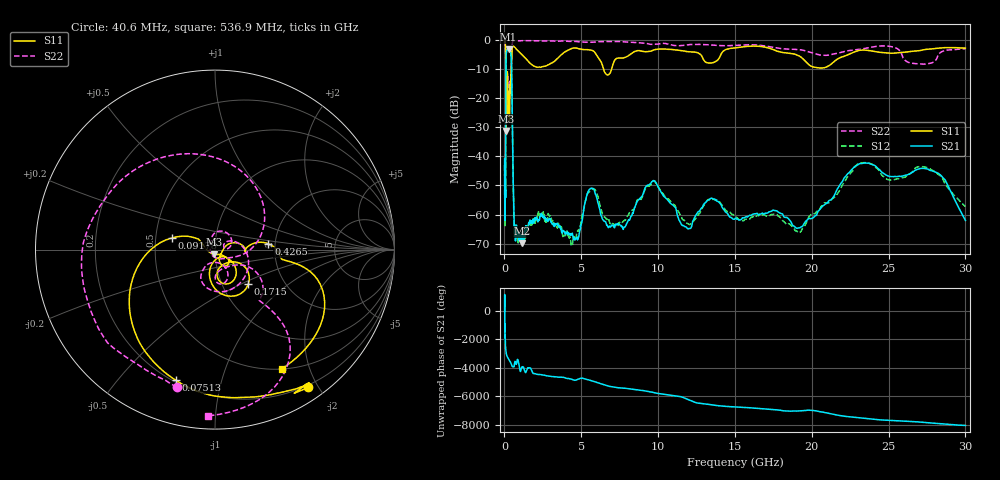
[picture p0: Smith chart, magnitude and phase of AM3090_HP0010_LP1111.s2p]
! Date/Time: Thu, Feb 28, 2019 1:56 PM
! Network Analyzer: Agilent Technologies E8364B Rev: A.07.50.67
! Sweep from 0.010 to 30.000 GHz, 1601 Points, Sweep Type: LOG
! Power Supply: 5.023 V, 0.002 A
# Hz S DB R 50
!freq MagS11 AngS11 MagS21 AngS21 MagS12 AngS12 MagS22 AngS22
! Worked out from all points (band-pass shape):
!   1601 points, 10 MHz to 30 GHz, reference 50 ohm
!   highest |S21| = -3.31 dB at 265.1 MHz (marker M1); lowest = -69.9 dB at 1.166 GHz (marker M2)
!   |S21| within 3 dB of the highest: 103.6 MHz to 441.7 MHz (338.1 MHz wide, 124 % of centre)
!   lowest |S11| = -31.3 dB at 99.92 MHz (marker M3), VSWR 1.06, Z = 49.5 - j2.64 ohm
!   |S11| at or under -10 dB: 90.68 MHz to 429.4 MHz (338.8 MHz wide, 130 % of centre); 6.451 GHz to 6.979 GHz (528.5 MHz wide, 7.87 % of centre)
!   |S22| runs from -31.6 to -0.2 dB; largest |S21 - S12| = 0.014
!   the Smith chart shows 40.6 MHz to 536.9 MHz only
!   S11 on the Smith chart (normalised r, x): 40.6 MHz: 0.17, -1.88; 75.13 MHz: 0.21, -0.72; 91.78 MHz: 0.61, +0.08; 171.5 MHz: 1.32, -0.55; 426.5 MHz: 1.84, +0.13; 536.9 MHz: 0.50, -1.59
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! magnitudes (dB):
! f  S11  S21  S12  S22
! 10 MHz  -0.3  -40.9  -43.0  -0.7
! 38.04 MHz  -0.5  -59.6  -60.0  -1.8
! 40.6 MHz  -0.7  -62.2  -62.2  -2.0
! 75.13 MHz  -2.4  -47.1  -48.2  -4.2
! 91.78 MHz  -12.0  -14.6  -14.7  -13.1
! 99.92 MHz  -31.3  -7.4  -7.4  -31.5
! 144.7 MHz  -19.2  -3.6  -3.6  -24.7
! 171.5 MHz  -11.5  -3.5  -3.5  -14.4
! 265.1 MHz  -21.2  -3.3  -3.3  -17.4
! 426.5 MHz  -10.5  -5.4  -5.4  -10.6
! 536.9 MHz  -2.4  -38.2  -38.1  -0.7
! 550.5 MHz  -2.3  -42.8  -42.7  -0.5
! 649.3 MHz  -2.4  -64.0  -67.7  -0.2
! 1.166 GHz  -5.2  -69.9  -66.3  -0.3
! 2.084 GHz  -9.4  -60.8  -61.7  -0.3
! 4.48 GHz  -2.8  -68.2  -67.7  -0.5
! 5.64 GHz  -3.5  -50.9  -51.7  -0.8
! 7.926 GHz  -5.9  -63.4  -61.4  -0.7
! 9.586 GHz  -3.7  -48.7  -49.2  -1.6
! 18.93 GHz  -5.0  -64.4  -65.6  -3.3
! 23.48 GHz  -3.5  -42.3  -42.2  -2.9
! 30 GHz  -2.9  -62.0  -57.3  -3.1
